| TEXAS INSTRUMENTS INCORPORATED
| Standard Linear and Logic Group
| IBIS Model of SN74ABT245B
| OCTAL BUS TRANSCEIVERS WITH 3-STATE OUTPUTS
| This file contains package information for the following:
|  PDIP 20-pin (N) package as [Component] ABT245B_N
|  QFN 20-pin (RGY) package as [Component] ABT245B_RGY
|  SOIC 20-pin (DW) package as [Component] ABT245B_DW
|  SOP 20-pin (NS) package as [Component] ABT245B_NS
|  SSOP 20-pin (DB) package as [Component] ABT245B_DB
|  TSSOP 20-pin (PW) package as [Component] ABT245B_PW
|  TVSOP 20-pin (DGV) package as [Component] ABT245B_DGV
|  VFBGA 20-pin (GQN) package as [Component] ABT245B_GQN
|  VFBGA 20-pin (ZQN) package as [Component] ABT245B_ZQN
| This device can be powered at the following Vccs:
|  5 volt Vcc
| This file provides unique models under the [Model Selector] for each Vcc.
| For operation at a specific Vcc, select the appropriate model after each
| [Model Selector] keyword.
[IBIS Ver]   3.2
[Comment char]  |_char
[File Name]   sn74abt245b.ibs
[File Rev]   1.1 | j_die
[Date]   April 20, 2005
[Source]   Data created from TI-SPICE simulations at TI-SLL.
[Notes]   The following is an IBIS list for the ABT245B.
   Please contact sllibis@ti.com with questions and
   comments concerning SLL IBIS models.
   This IBIS model is created from a BA (back annotated netlist)
   - FILE REV HISTORY
   - 1.1 Release IBIS file on 04/20/05
   - Non-monotonic data warning in pullup and pulldown
   is due to resistor at output.
   - Power clamp data deleted as there is no power-clamp diode.
[Disclaimer] Property of Texas Instruments Incorporated.  Unauthorized
   reproduction and/or distribution is strictly prohibited.
   This product is protected under copyright law.
   Created  2005, (C) Copyright  2005, Texas Instruments
   Incorporated, All Rights Reserved
   UNLESS THERE IS A SIGNED, WRITTEN AGREEMENT TO THE
   CONTRARY, TEXAS INSTRUMENTS (TI) IS PROVIDING THE IBIS
   MODELS  AND WITHOUT ANY WARRANTY, EXPRESSED OR
   IMPLIED.  TI assumes no liability for:
   1) the accuracy of the IBIS models provided to your
   company;
   2) the proper functioning of these IBIS Models in your
   design or for any resulting applications; or
   3) infringement of patents, copyrights or intellectual
   property rights resulting from your use of these IBIS
   models.
   TI provides IBIS Models as a service to our customers.
   You and your company shall not distribute, sell or give
   these models to anyone else without prior written
   permission from TI.
   TI reserves the right to make changes to our products or
   to discontinue any semiconductor product or service
   without notice, and advises our customers to obtain the
   latest version of relevant information to verify, before
   placing orders, that the information being relied on is
   current.
   Please be aware that your receipt and use of the IBIS
   information provided shall serve as acceptance of these
   terms and conditions.  If you do not accept these terms,
   you should return or destroy the IBIS models and any
   other accompanying information immediately.
| Component ABT245B_N 20-pin PDIP
[Component]   ABT245B_N
[Manufacturer]   Texas Instruments, Inc.
[Package]
|   typ   min   max
R_pkg   4.300e-02   3.800e-02   5.000e-02
L_pkg   7.384e-09   4.680e-09   1.032e-08
C_pkg   5.100e-13   2.310e-13   8.210e-13
[Pin]   signal_name   model_name   R_pin   L_pin   C_pin
1   DIR   ABT245B_DIR   4.200e-02   9.427e-09   8.100e-13
2   A1   ABT245B_AIO   4.600e-02   8.544e-09   4.560e-13
3   A2   ABT245B_AIO   4.800e-02   7.163e-09   4.350e-13
4   A3   ABT245B_AIO   4.000e-02   4.825e-09   2.610e-13
5   A4   ABT245B_AIO   4.000e-02   5.284e-09   6.480e-13
6   A5   ABT245B_AIO   4.000e-02   4.686e-09   2.320e-13
7   A6   ABT245B_AIO   4.000e-02   6.359e-09   4.890e-13
8   A7   ABT245B_AIO   3.800e-02   7.982e-09   4.750e-13
9   A8   ABT245B_AIO   4.300e-02   9.403e-09   4.750e-13
10   GND   GND   5.000e-02   1.032e-08   8.050e-13
11   B8   ABT245B_BIO   5.000e-02   1.028e-08   8.100e-13
12   B7   ABT245B_BIO   4.300e-02   9.383e-09   4.770e-13
13   B6   ABT245B_BIO   3.800e-02   7.978e-09   4.760e-13
14   B5   ABT245B_BIO   4.000e-02   6.302e-09   4.920e-13
15   B4   ABT245B_BIO   4.000e-02   4.680e-09   2.310e-13
16   B3   ABT245B_BIO   4.000e-02   5.284e-09   6.480e-13
17   B2   ABT245B_BIO   4.000e-02   4.822e-09   2.610e-13
18   B1   ABT245B_BIO   4.700e-02   7.118e-09   4.390e-13
19   NOE   ABT245B_NOE   4.600e-02   8.492e-09   4.610e-13
20   VCC   POWER   4.300e-02   9.348e-09   8.210e-13
| Component ABT245B_RGY 20-pin QFN
[Component]   ABT245B_RGY
[Manufacturer]   Texas Instruments, Inc.
[Package]
|   typ   min   max
R_pkg   5.000e-02   4.600e-02   5.500e-02
L_pkg   1.119e-09   1.025e-09   1.227e-09
C_pkg   3.520e-13   3.440e-13   3.630e-13
[Pin]   signal_name   model_name   R_pin   L_pin   C_pin
1   DIR   ABT245B_DIR   5.200e-02   1.167e-09   3.600e-13
2   A1   ABT245B_AIO   4.700e-02   1.049e-09   3.440e-13
3   A2   ABT245B_AIO   4.700e-02   1.055e-09   3.450e-13
4   A3   ABT245B_AIO   5.000e-02   1.119e-09   3.500e-13
5   A4   ABT245B_AIO   5.500e-02   1.227e-09   3.600e-13
6   A5   ABT245B_AIO   5.200e-02   1.167e-09   3.550e-13
7   A6   ABT245B_AIO   4.900e-02   1.087e-09   3.480e-13
8   A7   ABT245B_AIO   4.700e-02   1.054e-09   3.460e-13
9   A8   ABT245B_AIO   4.900e-02   1.091e-09   3.490e-13
10   GND   GND   5.300e-02   1.184e-09   3.620e-13
11   B8   ABT245B_BIO   5.300e-02   1.181e-09   3.600e-13
12   B7   ABT245B_BIO   5.000e-02   1.108e-09   3.490e-13
13   B6   ABT245B_BIO   4.800e-02   1.075e-09   3.470e-13
14   B5   ABT245B_BIO   5.000e-02   1.107e-09   3.490e-13
15   B4   ABT245B_BIO   5.400e-02   1.200e-09   3.620e-13
16   B3   ABT245B_BIO   5.100e-02   1.141e-09   3.570e-13
17   B2   ABT245B_BIO   4.700e-02   1.043e-09   3.440e-13
18   B1   ABT245B_BIO   4.600e-02   1.025e-09   3.440e-13
19   NOE   ABT245B_NOE   4.900e-02   1.090e-09   3.490e-13
20   VCC   POWER   5.400e-02   1.204e-09   3.630e-13
| Component ABT245B_DW 20-pin SOIC
[Component]   ABT245B_DW
[Manufacturer]   Texas Instruments, Inc.
[Package]
|   typ   min   max
R_pkg   3.800e-02   3.300e-02   4.500e-02
L_pkg   5.012e-09   4.110e-09   6.349e-09
C_pkg   7.170e-13   5.300e-13   8.680e-13
[Pin]   signal_name   model_name   R_pin   L_pin   C_pin
1   DIR   ABT245B_DIR   4.200e-02   6.336e-09   8.650e-13
2   A1   ABT245B_AIO   4.300e-02   5.542e-09   8.670e-13
3   A2   ABT245B_AIO   3.400e-02   4.714e-09   7.320e-13
4   A3   ABT245B_AIO   3.400e-02   4.377e-09   5.910e-13
5   A4   ABT245B_AIO   3.600e-02   4.130e-09   5.330e-13
6   A5   ABT245B_AIO   3.500e-02   4.111e-09   5.300e-13
7   A6   ABT245B_AIO   3.400e-02   4.284e-09   5.830e-13
8   A7   ABT245B_AIO   3.400e-02   4.634e-09   7.260e-13
9   A8   ABT245B_AIO   4.000e-02   5.518e-09   8.650e-13
10   GND   GND   4.300e-02   6.349e-09   8.660e-13
11   B8   ABT245B_BIO   4.100e-02   6.281e-09   8.610e-13
12   B7   ABT245B_BIO   4.500e-02   5.561e-09   8.680e-13
13   B6   ABT245B_BIO   3.300e-02   4.778e-09   7.420e-13
14   B5   ABT245B_BIO   3.500e-02   4.414e-09   5.960e-13
15   B4   ABT245B_BIO   3.500e-02   4.110e-09   5.330e-13
16   B3   ABT245B_BIO   3.600e-02   4.130e-09   5.330e-13
17   B2   ABT245B_BIO   3.400e-02   4.377e-09   5.910e-13
18   B1   ABT245B_BIO   3.400e-02   4.714e-09   7.310e-13
19   NOE   ABT245B_NOE   4.300e-02   5.569e-09   8.680e-13
20   VCC   POWER   4.200e-02   6.308e-09   8.640e-13
| Component ABT245B_NS 20-pin SOP
[Component]   ABT245B_NS
[Manufacturer]   Texas Instruments, Inc.
[Package]
|   typ   min   max
R_pkg   4.400e-02   2.900e-02   5.800e-02
L_pkg   3.666e-09   2.317e-09   5.115e-09
C_pkg   5.480e-13   3.160e-13   7.250e-13
[Pin]   signal_name   model_name   R_pin   L_pin   C_pin
1   DIR   ABT245B_DIR   5.800e-02   5.115e-09   7.250e-13
2   A1   ABT245B_AIO   5.300e-02   4.591e-09   7.240e-13
3   A2   ABT245B_AIO   4.900e-02   3.754e-09   5.720e-13
4   A3   ABT245B_AIO   2.900e-02   2.549e-09   3.880e-13
5   A4   ABT245B_AIO   3.100e-02   2.317e-09   3.160e-13
6   A5   ABT245B_AIO   3.100e-02   2.317e-09   3.160e-13
7   A6   ABT245B_AIO   2.900e-02   2.556e-09   3.990e-13
8   A7   ABT245B_AIO   4.900e-02   3.754e-09   5.790e-13
9   A8   ABT245B_AIO   5.300e-02   4.591e-09   7.240e-13
10   GND   GND   5.800e-02   5.115e-09   7.250e-13
11   B8   ABT245B_BIO   5.800e-02   5.115e-09   7.250e-13
12   B7   ABT245B_BIO   5.300e-02   4.591e-09   7.240e-13
13   B6   ABT245B_BIO   4.900e-02   3.754e-09   5.790e-13
14   B5   ABT245B_BIO   2.900e-02   2.557e-09   3.990e-13
15   B4   ABT245B_BIO   3.100e-02   2.317e-09   3.160e-13
16   B3   ABT245B_BIO   3.100e-02   2.317e-09   3.160e-13
17   B2   ABT245B_BIO   2.900e-02   2.557e-09   3.990e-13
18   B1   ABT245B_BIO   4.900e-02   3.754e-09   5.790e-13
19   NOE   ABT245B_NOE   5.300e-02   4.591e-09   7.240e-13
20   VCC   POWER   5.800e-02   5.115e-09   7.250e-13
| Component ABT245B_DB 20-pin SSOP
[Component]   ABT245B_DB
[Manufacturer]   Texas Instruments, Inc.
[Package]
|   typ   min   max
R_pkg   4.000e-02   3.500e-02   5.100e-02
L_pkg   3.495e-09   3.035e-09   4.314e-09
C_pkg   4.200e-13   3.460e-13   5.020e-13
[Pin]   signal_name   model_name   R_pin   L_pin   C_pin
1   DIR   ABT245B_DIR   4.900e-02   4.310e-09   5.020e-13
2   A1   ABT245B_AIO   4.800e-02   3.903e-09   4.870e-13
3   A2   ABT245B_AIO   3.500e-02   3.189e-09   3.960e-13
4   A3   ABT245B_AIO   3.500e-02   3.036e-09   3.470e-13
5   A4   ABT245B_AIO   3.500e-02   3.035e-09   3.670e-13
6   A5   ABT245B_AIO   3.500e-02   3.035e-09   3.670e-13
7   A6   ABT245B_AIO   3.500e-02   3.036e-09   3.470e-13
8   A7   ABT245B_AIO   3.500e-02   3.189e-09   3.970e-13
9   A8   ABT245B_AIO   4.700e-02   3.899e-09   4.880e-13
10   GND   GND   5.100e-02   4.314e-09   5.000e-13
11   B8   ABT245B_BIO   5.100e-02   4.314e-09   5.000e-13
12   B7   ABT245B_BIO   4.700e-02   3.899e-09   4.880e-13
13   B6   ABT245B_BIO   3.500e-02   3.189e-09   3.970e-13
14   B5   ABT245B_BIO   3.500e-02   3.036e-09   3.460e-13
15   B4   ABT245B_BIO   3.500e-02   3.035e-09   3.670e-13
16   B3   ABT245B_BIO   3.500e-02   3.035e-09   3.670e-13
17   B2   ABT245B_BIO   3.500e-02   3.036e-09   3.460e-13
18   B1   ABT245B_BIO   3.500e-02   3.189e-09   3.970e-13
19   NOE   ABT245B_NOE   4.700e-02   3.899e-09   4.880e-13
20   VCC   POWER   5.100e-02   4.314e-09   5.020e-13
| Component ABT245B_PW 20-pin TSSOP
[Component]   ABT245B_PW
[Manufacturer]   Texas Instruments, Inc.
[Package]
|   typ   min   max
R_pkg   5.000e-02   4.200e-02   6.000e-02
L_pkg   2.802e-09   2.248e-09   3.553e-09
C_pkg   3.170e-13   2.020e-13   4.430e-13
[Pin]   signal_name   model_name   R_pin   L_pin   C_pin
1   DIR   ABT245B_DIR   5.500e-02   3.461e-09   4.400e-13
2   A1   ABT245B_AIO   5.500e-02   3.150e-09   4.010e-13
3   A2   ABT245B_AIO   4.200e-02   2.619e-09   3.020e-13
4   A3   ABT245B_AIO   4.500e-02   2.273e-09   2.020e-13
5   A4   ABT245B_AIO   4.500e-02   2.248e-09   2.240e-13
6   A5   ABT245B_AIO   4.500e-02   2.273e-09   2.260e-13
7   A6   ABT245B_AIO   4.400e-02   2.323e-09   2.050e-13
8   A7   ABT245B_AIO   4.600e-02   2.704e-09   3.070e-13
9   A8   ABT245B_AIO   6.000e-02   3.265e-09   4.110e-13
10   GND   GND   5.700e-02   3.506e-09   4.360e-13
11   B8   ABT245B_BIO   5.800e-02   3.553e-09   4.370e-13
12   B7   ABT245B_BIO   5.800e-02   3.193e-09   4.050e-13
13   B6   ABT245B_BIO   4.200e-02   2.704e-09   3.110e-13
14   B5   ABT245B_BIO   4.600e-02   2.392e-09   2.100e-13
15   B4   ABT245B_BIO   4.700e-02   2.334e-09   2.290e-13
16   B3   ABT245B_BIO   4.700e-02   2.300e-09   2.270e-13
17   B2   ABT245B_BIO   4.700e-02   2.349e-09   2.070e-13
18   B1   ABT245B_BIO   4.500e-02   2.677e-09   3.060e-13
19   NOE   ABT245B_NOE   6.000e-02   3.235e-09   4.060e-13
20   VCC   POWER   5.600e-02   3.487e-09   4.430e-13
| Component ABT245B_DGV 20-pin TVSOP
[Component]   ABT245B_DGV
[Manufacturer]   Texas Instruments, Inc.
[Package]
|   typ   min   max
R_pkg   4.400e-02   3.800e-02   4.800e-02
L_pkg   2.561e-09   2.236e-09   2.961e-09
C_pkg   3.420e-13   2.640e-13   4.460e-13
[Pin]   signal_name   model_name   R_pin   L_pin   C_pin
1   DIR   ABT245B_DIR   4.400e-02   2.935e-09   4.170e-13
2   A1   ABT245B_AIO   4.200e-02   2.869e-09   4.460e-13
3   A2   ABT245B_AIO   4.300e-02   2.399e-09   3.160e-13
4   A3   ABT245B_AIO   4.400e-02   2.236e-09   2.650e-13
5   A4   ABT245B_AIO   4.600e-02   2.278e-09   2.640e-13
6   A5   ABT245B_AIO   4.500e-02   2.274e-09   2.640e-13
7   A6   ABT245B_AIO   4.400e-02   2.285e-09   2.690e-13
8   A7   ABT245B_AIO   4.300e-02   2.452e-09   3.200e-13
9   A8   ABT245B_AIO   4.400e-02   2.900e-09   4.460e-13
10   GND   GND   4.400e-02   2.961e-09   4.180e-13
11   B8   ABT245B_BIO   4.500e-02   2.954e-09   4.180e-13
12   B7   ABT245B_BIO   4.200e-02   2.847e-09   4.430e-13
13   B6   ABT245B_BIO   4.500e-02   2.453e-09   3.190e-13
14   B5   ABT245B_BIO   4.500e-02   2.297e-09   2.690e-13
15   B4   ABT245B_BIO   4.800e-02   2.334e-09   2.680e-13
16   B3   ABT245B_BIO   4.800e-02   2.335e-09   2.670e-13
17   B2   ABT245B_BIO   4.600e-02   2.299e-09   2.680e-13
18   B1   ABT245B_BIO   4.600e-02   2.457e-09   3.200e-13
19   NOE   ABT245B_NOE   4.300e-02   2.848e-09   4.410e-13
20   VCC   POWER   3.800e-02   2.812e-09   4.080e-13
| Component ABT245B_GQN 20-pin VFBGA
[Component]   ABT245B_GQN
[Manufacturer]   Texas Instruments, Inc.
[Package]
|   typ   min   max
R_pkg   4.300e-02   3.300e-02   6.100e-02
L_pkg   1.317e-09   8.960e-10   2.088e-09
C_pkg   1.130e-13   6.400e-14   1.900e-13
[Pin]   signal_name   model_name   R_pin   L_pin   C_pin
1   DIR   ABT245B_DIR   3.800e-02   1.199e-09   1.210e-13
2   A1   ABT245B_AIO   4.000e-02   1.067e-09   1.020e-13
3   A2   ABT245B_AIO   6.100e-02   1.999e-09   1.900e-13
4   A3   ABT245B_AIO   3.300e-02   9.630e-10   7.100e-14
5   A4   ABT245B_AIO   4.900e-02   1.523e-09   1.230e-13
6   A5   ABT245B_AIO   3.300e-02   8.960e-10   6.400e-14
7   A6   ABT245B_AIO   6.100e-02   1.899e-09   1.640e-13
8   A7   ABT245B_AIO   3.300e-02   8.980e-10   6.700e-14
9   A8   ABT245B_AIO   4.900e-02   1.514e-09   1.280e-13
10   GND   GND   3.600e-02   1.006e-09   9.400e-14
11   B8   ABT245B_BIO   4.900e-02   1.683e-09   1.460e-13
12   B7   ABT245B_BIO   3.300e-02   1.121e-09   8.900e-14
13   B6   ABT245B_BIO   6.100e-02   2.088e-09   1.730e-13
14   B5   ABT245B_BIO   3.300e-02   1.027e-09   7.100e-14
15   B4   ABT245B_BIO   4.900e-02   1.558e-09   1.240e-13
16   B3   ABT245B_BIO   3.300e-02   9.280e-10   6.700e-14
17   B2   ABT245B_BIO   6.100e-02   1.921e-09   1.770e-13
18   B1   ABT245B_BIO   3.300e-02   9.010e-10   7.700e-14
19   NOE   ABT245B_NOE   3.700e-02   9.900e-10   9.800e-14
20   VCC   POWER   3.500e-02   1.168e-09   1.190e-13
| Component ABT245B_ZQN 20-pin VFBGA
[Component]   ABT245B_ZQN
[Manufacturer]   Texas Instruments, Inc.
[Package]
|   typ   min   max
R_pkg   4.300e-02   3.300e-02   6.100e-02
L_pkg   1.317e-09   8.960e-10   2.088e-09
C_pkg   1.130e-13   6.400e-14   1.900e-13
[Pin]   signal_name   model_name   R_pin   L_pin   C_pin
1   DIR   ABT245B_DIR   3.800e-02   1.199e-09   1.210e-13
2   A1   ABT245B_AIO   4.000e-02   1.067e-09   1.020e-13
3   A2   ABT245B_AIO   6.100e-02   1.999e-09   1.900e-13
4   A3   ABT245B_AIO   3.300e-02   9.630e-10   7.100e-14
5   A4   ABT245B_AIO   4.900e-02   1.523e-09   1.230e-13
6   A5   ABT245B_AIO   3.300e-02   8.960e-10   6.400e-14
7   A6   ABT245B_AIO   6.100e-02   1.899e-09   1.640e-13
8   A7   ABT245B_AIO   3.300e-02   8.980e-10   6.700e-14
9   A8   ABT245B_AIO   4.900e-02   1.514e-09   1.280e-13
10   GND   GND   3.600e-02   1.006e-09   9.400e-14
11   B8   ABT245B_BIO   4.900e-02   1.683e-09   1.460e-13
12   B7   ABT245B_BIO   3.300e-02   1.121e-09   8.900e-14
13   B6   ABT245B_BIO   6.100e-02   2.088e-09   1.730e-13
14   B5   ABT245B_BIO   3.300e-02   1.027e-09   7.100e-14
15   B4   ABT245B_BIO   4.900e-02   1.558e-09   1.240e-13
16   B3   ABT245B_BIO   3.300e-02   9.280e-10   6.700e-14
17   B2   ABT245B_BIO   6.100e-02   1.921e-09   1.770e-13
18   B1   ABT245B_BIO   3.300e-02   9.010e-10   7.700e-14
19   NOE   ABT245B_NOE   3.700e-02   9.900e-10   9.800e-14
20   VCC   POWER   3.500e-02   1.168e-09   1.190e-13
| Models and submodels in the file (4): ABT245B_DIR (Input), ABT245B_NOE (Input), ABT245B_BIO (I/O), ABT245B_AIO (I/O)
